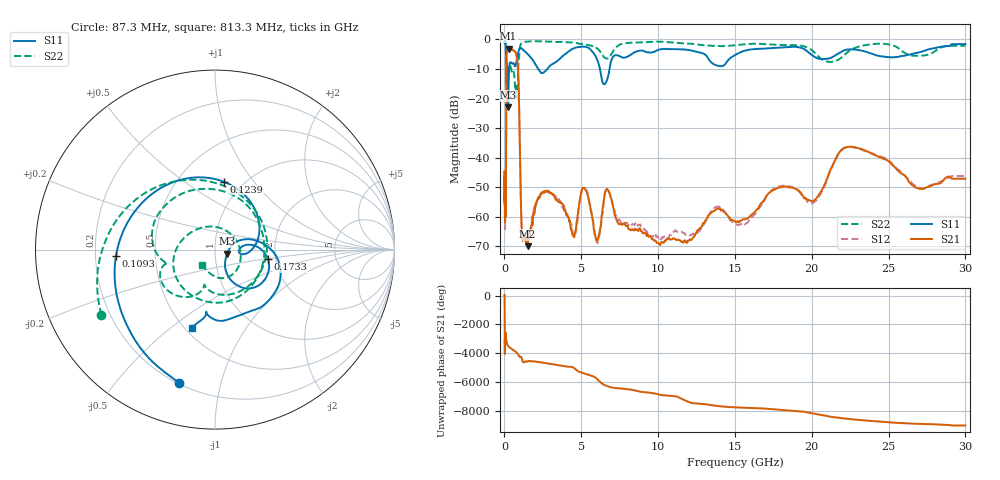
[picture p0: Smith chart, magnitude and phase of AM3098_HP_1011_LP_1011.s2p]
! Date/Time: Thu, Feb 28, 2019 8:43 AM
! Network Analyzer: Agilent Technologies E8364B Rev: A.07.50.67
! Sweep from 0.010 to 30.000 GHz, 1601 Points, Sweep Type: LOG
! Power Supply: 5.022 V, 0.001 A
# Hz S DB R 50
!freq MagS11 AngS11 MagS21 AngS21 MagS12 AngS12 MagS22 AngS22
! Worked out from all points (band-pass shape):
!   1601 points, 10 MHz to 30 GHz, reference 50 ohm
!   highest |S21| = -3.13 dB at 265.1 MHz (marker M1); lowest = -70.0 dB at 1.505 GHz (marker M2)
!   |S21| within 3 dB of the highest: 137.6 MHz to 807 MHz (669.4 MHz wide, 142 % of centre)
!   lowest |S11| = -23.0 dB at 242.3 MHz (marker M3), VSWR 1.15, Z = 57.2 - j2.55 ohm
!   |S11| at or under -10 dB: 191.7 MHz to 304.8 MHz (113.1 MHz wide, 45.5 % of centre); 2.194 GHz to 2.781 GHz (587.6 MHz wide, 23.6 % of centre); 6.219 GHz to 6.838 GHz (619.4 MHz wide, 9.49 % of centre)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
!   |S22| runs from -19.9 to -0.6 dB; largest |S21 - S12| = 0.011
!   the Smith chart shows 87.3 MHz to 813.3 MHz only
!   S11 on the Smith chart (normalised r, x): 87.3 MHz: 0.21, -0.74; 109.3 MHz: 0.29, -0.03; 123.9 MHz: 0.81, +0.72; 173.3 MHz: 1.82, -0.21; 813.3 MHz: 0.54, -0.59
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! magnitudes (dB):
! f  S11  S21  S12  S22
! 10 MHz  -0.4  -46.4  -46.0  -0.6
! 38.04 MHz  -0.4  -59.8  -60.1  -0.9
! 87.3 MHz  -2.3  -55.4  -53.7  -2.7
! 109.3 MHz  -5.1  -33.9  -33.7  -6.4
! 123.9 MHz  -8.4  -13.5  -13.5  -10.8
! 144.7 MHz  -17.3  -5.1  -5.0  -13.8
! 173.3 MHz  -10.5  -4.0  -4.0  -9.7
! 242.3 MHz  -23.0  -3.2  -3.1  -11.2
! 265.1 MHz  -16.0  -3.1  -3.1  -10.7
! 550.5 MHz  -8.1  -3.7  -3.6  -10.6
! 813.3 MHz  -6.9  -6.3  -6.3  -19.1
! 921.7 MHz  -3.9  -15.0  -14.9  -7.6
! 1.137 GHz  -3.1  -65.4  -63.8  -1.2
! 1.505 GHz  -4.9  -70.0  -66.5  -0.7
! 2.084 GHz  -9.0  -55.2  -55.2  -0.6
! 5.206 GHz  -2.4  -50.3  -50.3  -1.7
! 6.049 GHz  -7.1  -68.1  -69.0  -3.1
! 6.719 GHz  -13.0  -50.8  -50.8  -6.4
! 7.926 GHz  -6.0  -63.2  -62.0  -1.2
! 15.5 GHz  -4.0  -60.9  -62.0  -1.7
! 22.67 GHz  -3.4  -36.3  -36.5  -3.2
! 30 GHz  -1.6  -47.1  -46.2  -2.1
